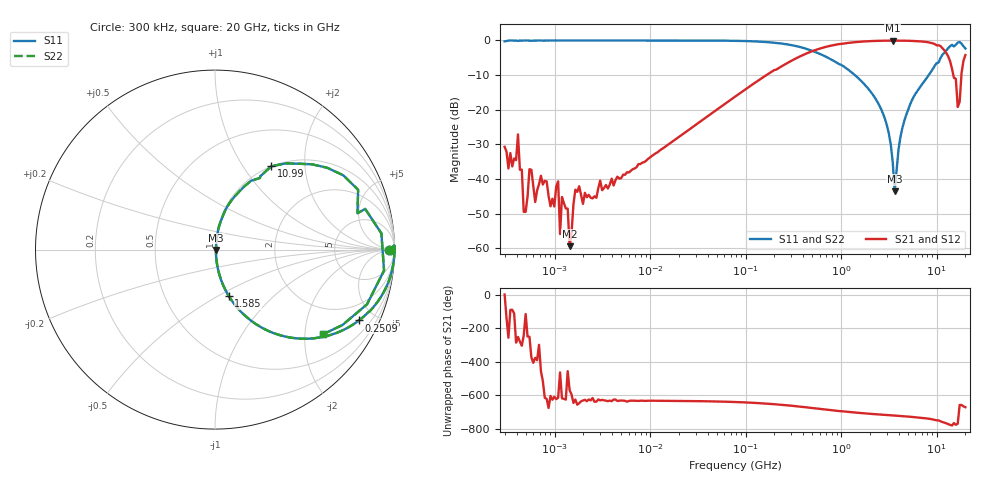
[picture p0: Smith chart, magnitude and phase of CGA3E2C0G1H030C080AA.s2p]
! S-parameter Generated by TDK Corporation
! Copyright(C) 2015 TDK Corporation.
! All Rights Reserved.
! TDK P/N: CGA3E2C0G1H030C080AA (Multilayer Ceramic Chip Capacitors)
! Property: C=3pF
! Size(LxWxT): 1.6x0.8x0.8mm, 0.063x0.031x0.031inches
! Model Type: s2p (Touchstone File Format Version 1.0)
! Frequency: DC=Yes Start=0.3MHz Stop=20000MHz 243points Log-sweep
! Note:
! Model Generated on Jun. 23, 2015
! Hash(MD5):
! Port Assignments:
!  1 ---| |--- 2
! Applicable Conditions:
!  Temperature = 25 degC
!  DC Bias Voltage = 0 V
!  Small Signal Operation
! Terms and conditions regarding TDK Simulation Models
! (1)This simulation model is being provided solely for informational purposes. Please refer to the specifications of the products in terms of detailed characteristics of such products.
! (2)In no event shall TDK Corporation of any of its subsidiaries be liable for any loss or damage arising, directly or indirectly,
!  From any information contained in this simulation model, including, but not limited to loss or damages arising from any inaccuracies, omissions or errors in connection with such information.
! (3)Any and all copyrights on this simulation model are owned by TDK Corporation.
!  Duplication or redistribution of this simulation model without prior written permission from TDK Corporation is prohibited.
! (4)This simulation model is subject to any modification or change without any prior notice.
! (5)Neither TDK Corporation nor any of its subsidiaries shall make any warranty, express or implied,
!  Including but not limited to the correctness, implied warranties of merchantability and fitness for a particular purpose with respect to this simulation models.
! (6)The use of this simulation model shall be deemed to have consented to the terms and conditions hereof.
# MHz S MA R 50
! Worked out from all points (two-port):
!   242 points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, 300 kHz to 20 GHz, reference 50 ohm
!   highest |S21| = -0.05 dB at 3.471 GHz (marker M1); lowest = -59.4 dB at 1.438 MHz (marker M2)
!   |S21| within 3 dB of the highest: 503 MHz to 12.2 GHz (11.7 GHz wide, 184 % of centre)
!   lowest |S11| = -43.6 dB at 3.634 GHz (marker M3), VSWR 1.01, Z = 50.6 - j0.212 ohm
!   |S11| at or under -10 dB: 1.393 GHz to 8.262 GHz (6.868 GHz wide, 142 % of centre)
!   |S22| runs from -43.6 to 0.0 dB; largest |S21 - S12| = 1e-14
!   S11 on the Smith chart (normalised r, x): 300 kHz: 68, -2; 250.9 MHz: 1.03, -4.05; 1.585 GHz: 1.01, -0.56; 10.99 GHz: 1.00, +1.35; 20 GHz: 1.09, -2.48
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0.3  0.9709 -0.0  0.02916 1.5  0.02916 1.5  0.9709 -0.0
0.4142236  0.9837 -1.5  0.04404 109.0  0.04404 109.0  0.9837 -1.5
0.4756456  0.9984 -0.0  0.003356 118.3  0.003356 118.3  0.9984 -0.0
0.5461754  0.9951 -0.7  0.01387 109.7  0.01387 109.7  0.9951 -0.7
1.090374  0.9973 -0.4  0.009259 106.3  0.009259 106.3  0.9973 -0.4
1.141804  0.9996 0.0  0.001607 -102.7  0.001607 -102.7  0.9996 0.0
1.19566  0.9987 -0.3  0.005507 102.8  0.005507 102.8  0.9987 -0.3
1.437715  0.9991 -0.0  0.001074 151.6  0.001074 151.6  0.9991 -0.0
1.650902  0.9992 -0.4  0.007022 95.8  0.007022 95.8  0.9992 -0.4
1.985118  1 -0.2  0.004373 90.2  0.004373 90.2  1 -0.2
12.54397  0.9996 -1.5  0.02565 88.3  0.02565 88.3  0.9996 -1.5
79.26541  0.9875 -9.1  0.1577 80.9  0.1577 80.9  0.9875 -9.1
250.8934  0.8939 -26.2  0.4413 63.4  0.4413 63.4  0.8939 -26.2
500.8786  0.7069 -44.6  0.7026 45.0  0.7026 45.0  0.7069 -44.6
1585.397  0.2686 -73.5  0.959 15.6  0.959 15.6  0.2686 -73.5
3165.055  0.04496 -81.1  0.994 2.6  0.994 2.6  0.04496 -81.1
3470.673  0.0175 -71.1  0.9945 1.0  0.9945 1.0  0.0175 -71.1
3634.376  0.006629 -18.4  0.9937 0.1  0.9937 0.1  0.006629 -18.4
4792.115  0.08357 81.3  0.9908 -4.8  0.9908 -4.8  0.08357 81.3
10985.48  0.5598 56.0  0.8284 -34.1  0.8284 -34.1  0.5598 56.0
16632.79  0.9314 5.6  0.1096 -48.2  0.1096 -48.2  0.9314 5.6
20000  0.7655 -38.0  0.6161 49.9  0.6161 49.9  0.7655 -38.0
